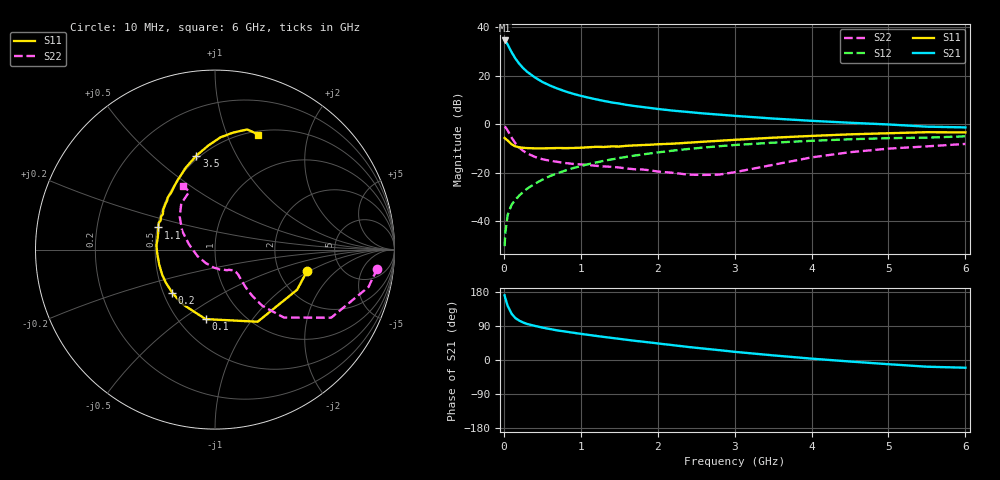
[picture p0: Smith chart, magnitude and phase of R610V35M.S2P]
! SIEMENS Small Signal Semiconductors
! BFR193
! Si NPN RF Bipolar Junction Transistor in SOT23
! VCE = 10 V  IC = 35 mA
! Common Emitter S-Parameters:  May  1996
# GHz  S  MA  R  50
!  f  S11  S21  S12  S22
! GHz  MAG  ANG  MAG  ANG  MAG  ANG  MAG  ANG
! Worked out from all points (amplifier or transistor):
!   36 points, 10 MHz to 6 GHz, reference 50 ohm
!   highest |S21| = 34.6 dB at 10 MHz (marker M1)
!   |S21| within 3 dB of that: start of sweep to 71.17 MHz
!   unconditionally stable (mu >= 1): 490.7 MHz to 2.23 GHz
!   at 250 MHz: K = 0.89, MSG = 25.5 dB, |S12| = -27.8 dB
!   at 1.4 GHz: K = 1.02, MAG = 10.8 dB, |S12| = -14.4 dB
!   at 6 GHz: K = 0.94, MSG = 1.8 dB, |S12| = -4.9 dB
!   S11 on the Smith chart (normalised r, x): 10 MHz: 2.89, -0.94; 100 MHz: 0.67, -0.62; 200 MHz: 0.56, -0.30; 1.1 GHz: 0.51, +0.14; 3.5 GHz: 0.48, +0.70; 6 GHz: 0.54, +1.30
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0.01  0.5271 -12.9  53.91 170.7  0.0031 78.4  0.9107 -6.7
0.02  0.5095 -26.0  52.45 162.5  0.006 77.5  0.88 -13.7
0.05  0.4669 -59.4  44.35 142.6  0.0137 69.4  0.7501 -30.4
0.1  0.3908 -97.7  31.11 122.3  0.022 64.8  0.539 -44.6
0.15  0.3536 -121.5  22.91 110.6  0.0281 64.7  0.4093 -49.9
0.2  0.3379 -134.9  17.92 103.9  0.0342 66.9  0.335 -51.1
0.25  0.3302 -145.8  14.57 99.0  0.0406 67.5  0.2867 -51.1
0.3  0.3261 -154.3  12.3 95.3  0.0471 69.2  0.2554 -50.4
0.4  0.3219 -164.8  9.403 90.2  0.0597 70.6  0.216 -48.8
0.5  0.3214 -173.0  7.541 85.6  0.0727 70.7  0.1922 -47.3
0.6  0.3239 -179.3  6.338 81.7  0.0863 70.8  0.1789 -46.9
0.8  0.3253 170.5  4.8 75.0  0.1123 69.3  0.1605 -47.6
0.9  0.3274 166.4  4.291 72.0  0.1258 68.8  0.1538 -47.9
1.1  0.3391 158.7  3.573 66.3  0.1522 66.6  0.1458 -51.8
1.3  0.3437 151.8  3.056 60.9  0.1778 64.1  0.1364 -55.8
1.6  0.3633 142.5  2.527 53.2  0.2157 60.2  0.1235 -65.5
2.2  0.4016 127.2  1.927 39.1  0.2892 51.9  0.1008 -93.5
2.8  0.4607 113.6  1.595 26.0  0.3563 42.9  0.0926 -142.7
3.5  0.5338 101.2  1.325 12.2  0.4214 32.1  0.1474 168.8
4.5  0.6257 87.3  1.085 -4.0  0.4952 18.4  0.2682 137.1
5.5  0.6929 75.0  0.901 -17.7  0.5354 4.7  0.3536 113.9
6  0.6852 69.3  0.87 -20.4  0.5694 0.9  0.3971 116.5
